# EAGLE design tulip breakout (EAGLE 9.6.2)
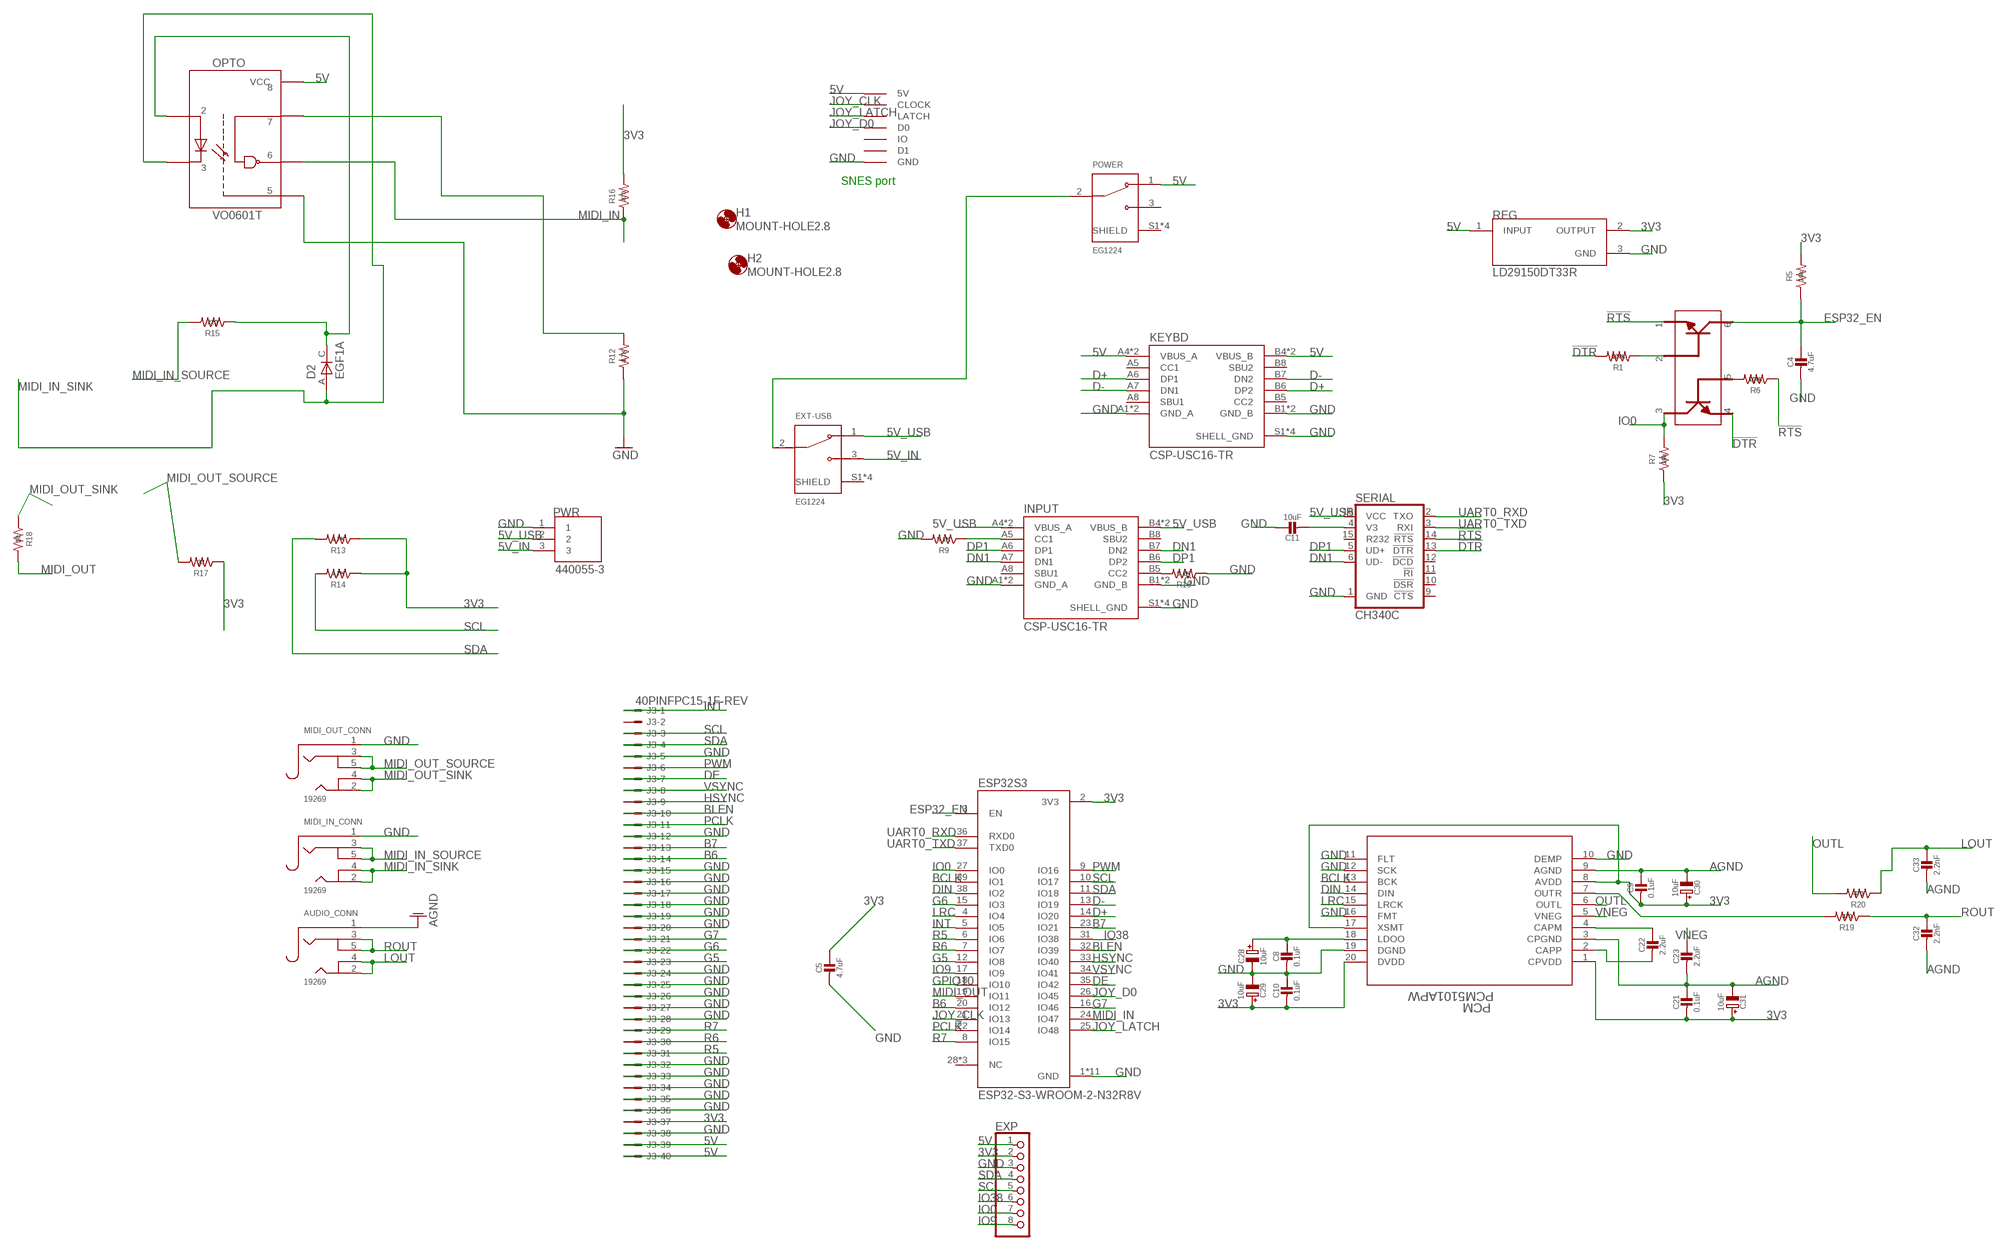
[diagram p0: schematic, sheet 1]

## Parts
AUDIO_CONN  19269  AUDIO_3.5MMJACK  [4UCONN_19269]
C4  4.7uF  CAP_CERAMIC0805-NOOUTLINE  [0805-NO]
C5  4.7uF  CAP_CERAMIC0805-NOOUTLINE  [0805-NO]
C8  0.1uF  CAP_CERAMIC0805-NOOUTLINE  [0805-NO]
C9  0.1uF  CAP_CERAMIC0805-NOOUTLINE  [0805-NO]
C10  0.1uF  CAP_CERAMIC0805-NOOUTLINE  [0805-NO]
C11  10uF  CAP_CERAMIC0805-NOOUTLINE  [0805-NO]
C21  0.1uF  CAP_CERAMIC0805-NOOUTLINE  [0805-NO]
C22  2.2uF  CAP_CERAMIC0805-NOOUTLINE  [0805-NO]
C23  2.2uF  CAP_CERAMIC0805-NOOUTLINE  [0805-NO]
C28  10uF  CAP_ELECTROLYTICPANASONIC_C  [PANASONIC_C]
C29  10uF  CAP_ELECTROLYTICPANASONIC_C  [PANASONIC_C]
C30  10uF  CAP_ELECTROLYTICPANASONIC_C  [PANASONIC_C]
C31  10uF  CAP_ELECTROLYTICPANASONIC_C  [PANASONIC_C]
C32  2.2nF  CAP_CERAMIC0805-NOOUTLINE  [0805-NO]
C33  2.2nF  CAP_CERAMIC0805-NOOUTLINE  [0805-NO]
D2  EGF1A  [DIOM449X264X300L114X135N]
ESP32S3  ESP32-S3-WROOM-2-N32R8V  [XCVR_ESP32-S3-WROOM-2-N32R8V]
EXP  PINHD-1X8BIG  [1X08-BIG]
EXT-USB  EG1224  [SW_EG1224]
H1  MOUNT-HOLE2.8  [2,8]
H2  MOUNT-HOLE2.8  [2,8]
INPUT  CSP-USC16-TR  [VALCON_CSP-USC16-TR]
J3  40PINFPC15-1F-REV  [XF2M-4015-1F-REVERSE]
KEYBD  CSP-USC16-TR  [VALCON_CSP-USC16-TR]
MIDI_IN_CONN  19269  AUDIO_3.5MMJACK  [4UCONN_19269]
MIDI_OUT_CONN  19269  AUDIO_3.5MMJACK  [4UCONN_19269]
OPTO  VO0601T  [SOIC127P610X331-8N]
PCM  PCM5101APW  [PW20_TEX]
POWER  EG1224  [SW_EG1224]
PWR  440055-3  [TE_440055-3]
R1  100k  R-US_R0805  [R0805]
R5  10k  R-US_R0805  [R0805]
R6  100k  R-US_R0805  [R0805]
R7  10k  R-US_R0805  [R0805]
R9  5.1K  R-US_R0805  [R0805]
R10  5.1K  R-US_R0805  [R0805]
R12  4.7K  R-US_R0805  [R0805]
R13  4.7K  R-US_R0805  [R0805]
R14  4.7K  R-US_R0805  [R0805]
R15  220  R-US_R0805  [R0805]
R16  470  R-US_R0805  [R0805]
R17  33  R-US_R0805  [R0805]
R18  10  R-US_R0805  [R0805]
R19  470  R-US_R0805  [R0805]
R20  470  R-US_R0805  [R0805]
REG  LD29150DT33R  [DPAK456P972X240-3N]
RESET  MBT3904DW1T1G  [SOT236]
SERIAL  CH340C  [SO016]
SNES  SNESCONN  [SNESCONN]

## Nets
3V3: C5.1 C9.2 C10.2 C21.2 C29.+ C30.+ C31.+ ESP32S3.2(3V3) EXP.2 J3.37 PCM.1(CPVDD) PCM.8(AVDD) PCM.17(XSMT) PCM.20(DVDD) R5.2 R7.1 R13.1 R14.1 R16.2 R17.1 REG.2(OUTPUT)
5V: EXP.1 J3.39 J3.40 KEYBD.A4(VBUS_A) KEYBD.A9(VBUS_A) KEYBD.B4(VBUS_B) KEYBD.B9(VBUS_B) OPTO.8(VCC) POWER.1 REG.1(INPUT) SNES.5V
5V_IN: EXT-USB.3 PWR.3
5V_USB: EXT-USB.1 INPUT.A4(VBUS_A) INPUT.A9(VBUS_A) INPUT.B4(VBUS_B) INPUT.B9(VBUS_B) PWR.2 SERIAL.16(VCC)
!DTR: R1.2 RESET.4 SERIAL.13(!DTR)
!RTS: R6.1 RESET.1 SERIAL.14(!RTS)
AGND: AUDIO_CONN.1 C9.1 C21.1 C23.2 C30.- C31.- C32.2 C33.2 PCM.3(CPGND) PCM.9(AGND)
B6: ESP32S3.20(IO12) J3.14
B7: ESP32S3.23(IO21) J3.13
BCLK: ESP32S3.39(IO1) PCM.13(BCK)
BLEN: ESP32S3.32(IO39) J3.10
D+: ESP32S3.14(IO20) KEYBD.A6(DP1) KEYBD.B6(DP2)
D-: ESP32S3.13(IO19) KEYBD.A7(DN1) KEYBD.B7(DN2)
DE: ESP32S3.35(IO42) J3.7
DIN: ESP32S3.38(IO2) PCM.14(DIN)
DN1: INPUT.A7(DN1) INPUT.B7(DN2) SERIAL.6(UD-)
DP1: INPUT.A6(DP1) INPUT.B6(DP2) SERIAL.5(UD+)
ESP32_EN: C4.1 ESP32S3.3(EN) R5.1 RESET.6
EXT-USB: EXT-USB.2 POWER.2
G5: ESP32S3.12(IO8) J3.23
G6: ESP32S3.15(IO3) J3.22
G7: ESP32S3.16(IO46) J3.21
GND: C4.2 C5.2 C8.2 C10.1 C11.1 C28.- C29.- ESP32S3.1(GND) ESP32S3.40(GND) ESP32S3.41_1(GND) ESP32S3.41_2(GND) ESP32S3.41_3(GND) ESP32S3.41_4(GND) ESP32S3.41_5(GND) ESP32S3.41_6(GND) ESP32S3.41_7(GND) ESP32S3.41_8(GND) ESP32S3.41_9(GND) EXP.3 INPUT.A1(GND_A) INPUT.A12(GND_A) INPUT.B1(GND_B) INPUT.B12(GND_B) INPUT.S1(SHELL_GND) INPUT.S2(SHELL_GND) INPUT.S3(SHELL_GND) INPUT.S4(SHELL_GND) J3.5 J3.12 J3.15 J3.16 J3.17 J3.18 J3.19 J3.20 J3.24 J3.25 J3.26 J3.27 J3.28 J3.32 J3.33 J3.34 J3.35 J3.36 J3.38 KEYBD.A1(GND_A) KEYBD.A12(GND_A) KEYBD.B1(GND_B) KEYBD.B12(GND_B) KEYBD.S1(SHELL_GND) KEYBD.S2(SHELL_GND) KEYBD.S3(SHELL_GND) KEYBD.S4(SHELL_GND) MIDI_IN_CONN.1 MIDI_OUT_CONN.1 OPTO.5(GND) PCM.10(DEMP) PCM.11(FLT) PCM.12(SCK) PCM.16(FMT) PCM.19(DGND) PWR.1 R9.2 R10.1 R12.1 REG.3(GND) SERIAL.1(GND) SNES.GND
GPIO10: ESP32S3.18(IO10)
HSYNC: ESP32S3.33(IO40) J3.9
INT: ESP32S3.5(IO5) J3.1
IO0: ESP32S3.27(IO0) EXP.7 R7.2 RESET.3
IO9: ESP32S3.17(IO9) EXP.8
IO38: ESP32S3.31(IO38) EXP.6
JOY_CLK: ESP32S3.21(IO13) SNES.CLOCK
JOY_D0: ESP32S3.26(IO45) SNES.D0
JOY_LATCH: ESP32S3.25(IO48) SNES.LATCH
LOUT: AUDIO_CONN.2 AUDIO_CONN.4 C33.1 R20.1
LRC: ESP32S3.4(IO4) PCM.15(LRCK)
MIDI_IN: ESP32S3.24(IO47) OPTO.6(VO) R16.1
MIDI_IN_SINK: D2.A MIDI_IN_CONN.2 MIDI_IN_CONN.4 OPTO.3(C)
MIDI_IN_SOURCE: MIDI_IN_CONN.3 MIDI_IN_CONN.5 R15.2
MIDI_OUT: ESP32S3.19(IO11) R18.2
MIDI_OUT_SINK: MIDI_OUT_CONN.2 MIDI_OUT_CONN.4 R18.1
MIDI_OUT_SOURCE: MIDI_OUT_CONN.3 MIDI_OUT_CONN.5 R17.2
N$1: R1.1 RESET.2
N$2: R6.2 RESET.5
N$3: INPUT.B5(CC2) R10.2
N$7: C8.1 C28.+ PCM.18(LDOO)
N$8: PCM.7(OUTR) R19.2
N$16: C22.1 PCM.4(CAPM)
N$18: C22.2 PCM.2(CAPP)
N$30: D2.C OPTO.2(A) R15.1
N$32: OPTO.7(VE) R12.2
N$38: C11.2 SERIAL.4(V3)
N$42: INPUT.A5(CC1) R9.1
OUTL: PCM.6(OUTL) R20.2
PCLK: ESP32S3.22(IO14) J3.11
PWM: ESP32S3.9(IO16) J3.6
R5: ESP32S3.6(IO6) J3.31
R6: ESP32S3.7(IO7) J3.30
R7: ESP32S3.8(IO15) J3.29
ROUT: AUDIO_CONN.3 AUDIO_CONN.5 C32.1 R19.1
SCL: ESP32S3.10(IO17) EXP.5 J3.3 R14.2
SDA: ESP32S3.11(IO18) EXP.4 J3.4 R13.2
UART0_RXD: ESP32S3.36(RXD0) SERIAL.2(TXO)
UART0_TXD: ESP32S3.37(TXD0) SERIAL.3(RXI)
VNEG: C23.1 PCM.5(VNEG)
VSYNC: ESP32S3.34(IO41) J3.8
Unconnected: ESP32S3.28(NC) ESP32S3.29(NC) ESP32S3.30(NC) EXT-USB.S1(SHIELD) EXT-USB.S2(SHIELD) EXT-USB.S3(SHIELD) EXT-USB.S4(SHIELD) INPUT.A8(SBU1) INPUT.B8(SBU2) J3.2 KEYBD.A5(CC1) KEYBD.A8(SBU1) KEYBD.B5(CC2) KEYBD.B8(SBU2) POWER.3 POWER.S1(SHIELD) POWER.S2(SHIELD) POWER.S3(SHIELD) POWER.S4(SHIELD) SERIAL.9(!CTS) SERIAL.10(!DSR) SERIAL.11(!RI) SERIAL.12(!DCD) SERIAL.15(R232) SNES.D1 SNES.IO

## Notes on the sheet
- SNES port

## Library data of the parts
AUDIO_CONN MIDI_IN_CONN MIDI_OUT_CONN = microbuilder:AUDIO_3.5MMJACK: 3.5MM Audio Jack These are normally connected as follows, from left-to right on the schematic symbol above: Tip: Left Audio Inner Ring: Right Audio Shell: Common/GND
C4 C5 C8-C11 C21-C23 C32 C33 = microbuilder:CAP_CERAMIC: Ceramic Capacitors
C28-C31 = microbuilder:CAP_ELECTROLYTIC: Electrolytic Capacitors
D2 = EGF1A:EGF1A: EGF1A Series 1 A 100 V 50 ns Surface Mount Fast Recovery Rectifier - DO-214AC Check availability; AVAILABILITY: In Stock; DESCRIPTION: Diode Standard 50 V 1A Surface Mount DO-214AC (SMA); MF: ON Semiconductor; MP: EGF1A; PACKAGE: SMA-2 ON Semiconductor; PRICE: None; PURCHASE-URL: https://pricing.snapeda.com/search/part/EGF1A/?ref=eda
ESP32S3 = ESP32-S3-WROOM-2-N32R8V:ESP32-S3-WROOM-2-N32R8V: Check availability; AVAILABILITY: In Stock; DESCRIPTION: Bluetooth, WiFi 802.11b/g/n, Bluetooth v5.0 Transceiver Module 2.4GHz PCB Trace Surface Mount; MF: Espressif Systems; MP: ESP32-S3-WROOM-2-N32R8V; PACKAGE: Package; PRICE: None; PURCHASE-URL: https://pricing.snapeda.com/search/part/ESP32-S3-WROOM-2-N32R8V/?ref=eda
EXP = adafruit:PINHD-1X8: PIN HEADER
EXT-USB POWER = EG1224:EG1224; DESCRIPTION: Slide Switch SPDT Through Hole, Right Angle; DIGI-KEY_PART_NUMBER: EG2585-ND; MF: E-Switch; MP: EG1224; PACKAGE: None; PURCHASE-URL: https://pricing.snapeda.com/search/part/EG1224/?ref=eda
H1 H2 = holes:MOUNT-HOLE: MOUNTING HOLE with drill center marker
INPUT KEYBD = CSP-USC16-TR:CSP-USC16-TR: CSP-USC16-TR Valcon USB Type C Surface Mount PCB Socket Check availability; AVAILABILITY: In Stock; DESCRIPTION: CSP-USC16-TR Valcon USB Type C Surface Mount PCB Socket; MF: Valcon; MP: CSP-USC16-TR; PACKAGE: None; PRICE: None; PURCHASE-URL: https://pricing.snapeda.com/search/part/CSP-USC16-TR/?ref=eda
J3 = adafruit:40PINFPC: OMRON FPC Connector Source : http://www.omron.com/ecb/products/pdf/fpc.pdf XF2M-4015-rev is good for connecting up 'PSP' SHARP LQ043 LCDs
OPTO = VO0601T:VO0601T: High Speed Optocoupler, 10 MBd, SOIC-8 Package; DESCRIPTION: Logic Output Optoisolator 10MBd Open Drain 4000Vrms 1 Channel 5kV/µs CMTI 8-SOIC; DIGI-KEY_PART_NUMBER: 751-1377-2-ND; MF: Vishay Semiconductors; MP: VO0601T; PACKAGE: None; PURCHASE-URL: https://pricing.snapeda.com/search/part/VO0601T/?ref=eda
PCM = pcm5101apw:PCM5101APW; COPYRIGHT: Copyright (C) 2022 Ultra Librarian. All rights reserved.; DIGI-KEY_PART_NUMBER_1: PCM5101APW-ND; MANUFACTURER_PART_NUMBER: PCM5101APW; MFR_NAME: Texas Instruments
PWR = 440055-3:440055-3; COMMENT: 440055-3; DESCRIPTION: Connector Header Through Hole, Right Angle 3 position 0.079 (2.00mm); DIGI-KEY_PART_NUMBER: A100044-ND; EU_ROHS_COMPLIANCE: Compliant; MF: TE Connectivity; MP: 440055-3; PACKAGE: None; PURCHASE-URL: https://pricing.snapeda.com/search/part/440055-3/?ref=eda
R1 R5-R7 R9 R10 R12-R20 = adafruit:R-US_: RESISTOR, American symbol
REG = LD29150DT33R:LD29150DT33R: LD29150 Series 1.5 A 3.3 V Fixed Output SMT LDO Voltage Regulator - TO-252; DESCRIPTION: Linear Voltage Regulator IC Positive Fixed 1 Output 1.5A DPAK; DIGI-KEY_PART_NUMBER: 497-1496-2-ND; MF: STMicroelectronics; MP: LD29150DT33R; PACKAGE: TO-252 STMicroelectronics; PURCHASE-URL: https://pricing.snapeda.com/search/part/LD29150DT33R/?ref=eda
RESET = MBT3904DW1T1G:MBT3904DW1T1G: Check availability; AVAILABILITY: In Stock; DESCRIPTION: Bipolar (BJT) Transistor Array 2 NPN (Dual) 40V 200mA 300MHz 150mW Surface Mount SC-88/SC70-6/SOT-363; MF: ON Semiconductor; MP: MBT3904DW1T1G; PACKAGE: SC-88-6 ON Semiconductor; PRICE: None; PURCHASE-URL: https://pricing.snapeda.com/search/part/MBT3904DW1T1G/?ref=eda
SERIAL = SparkFun-IC-Comms:CH340C; PROD_ID: IC-14038
SNES = gamepad-conn:SNESCONN

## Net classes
1 power: width 0.178 mm

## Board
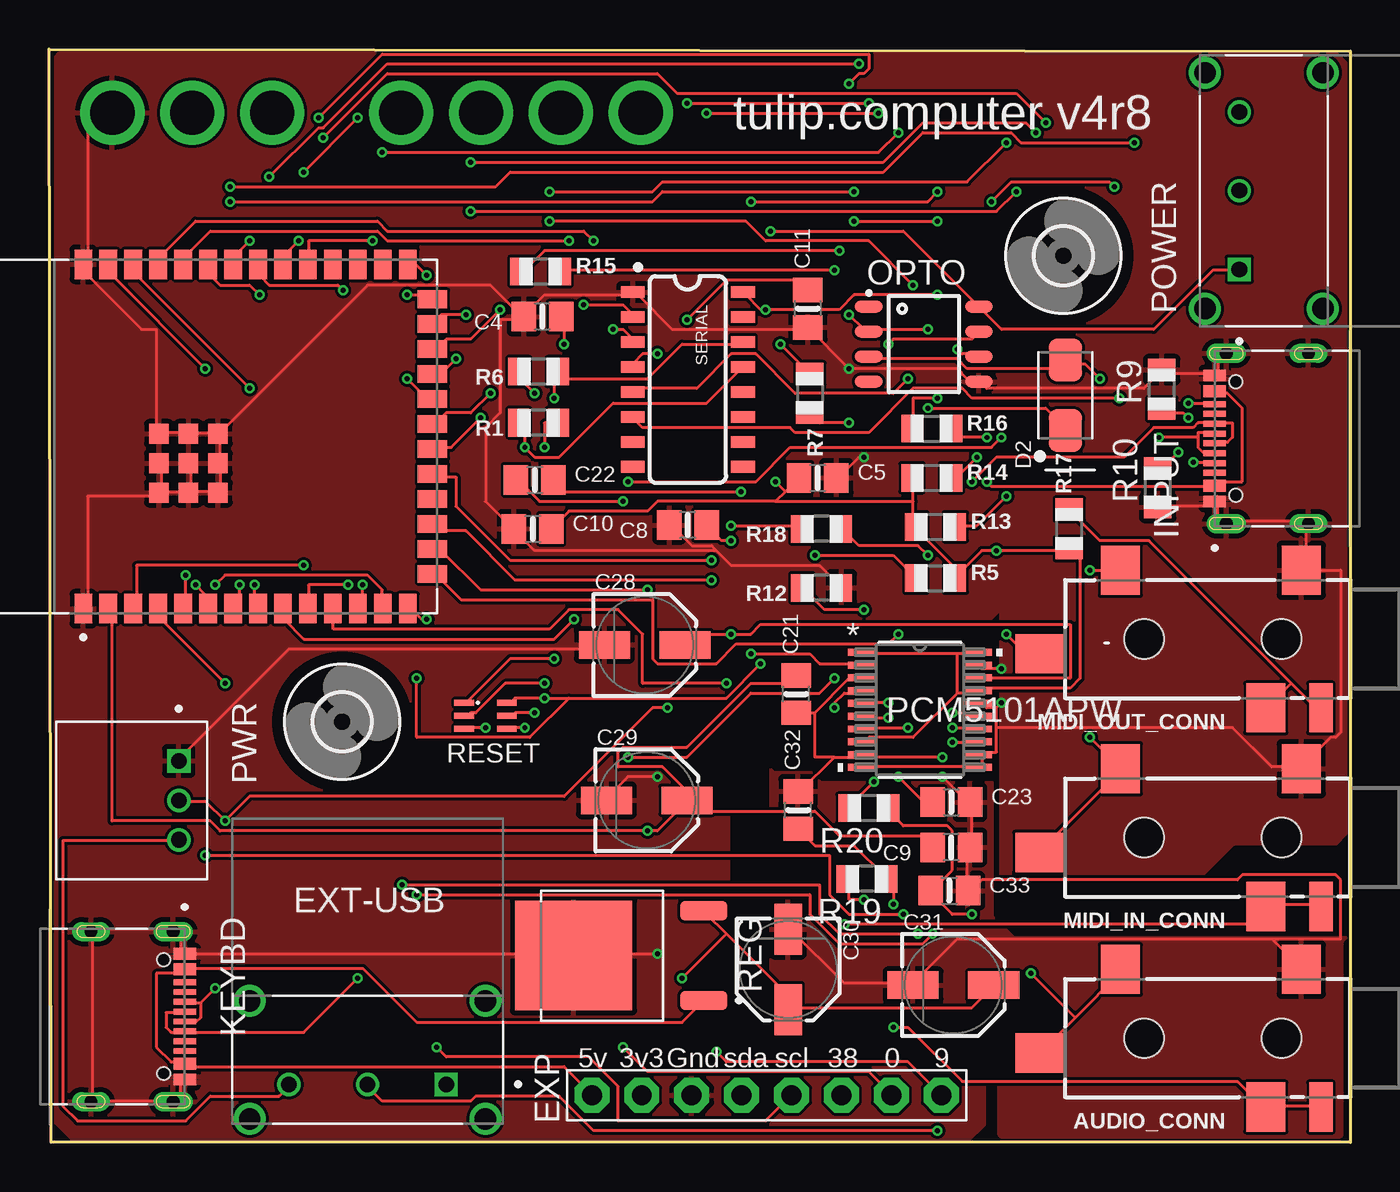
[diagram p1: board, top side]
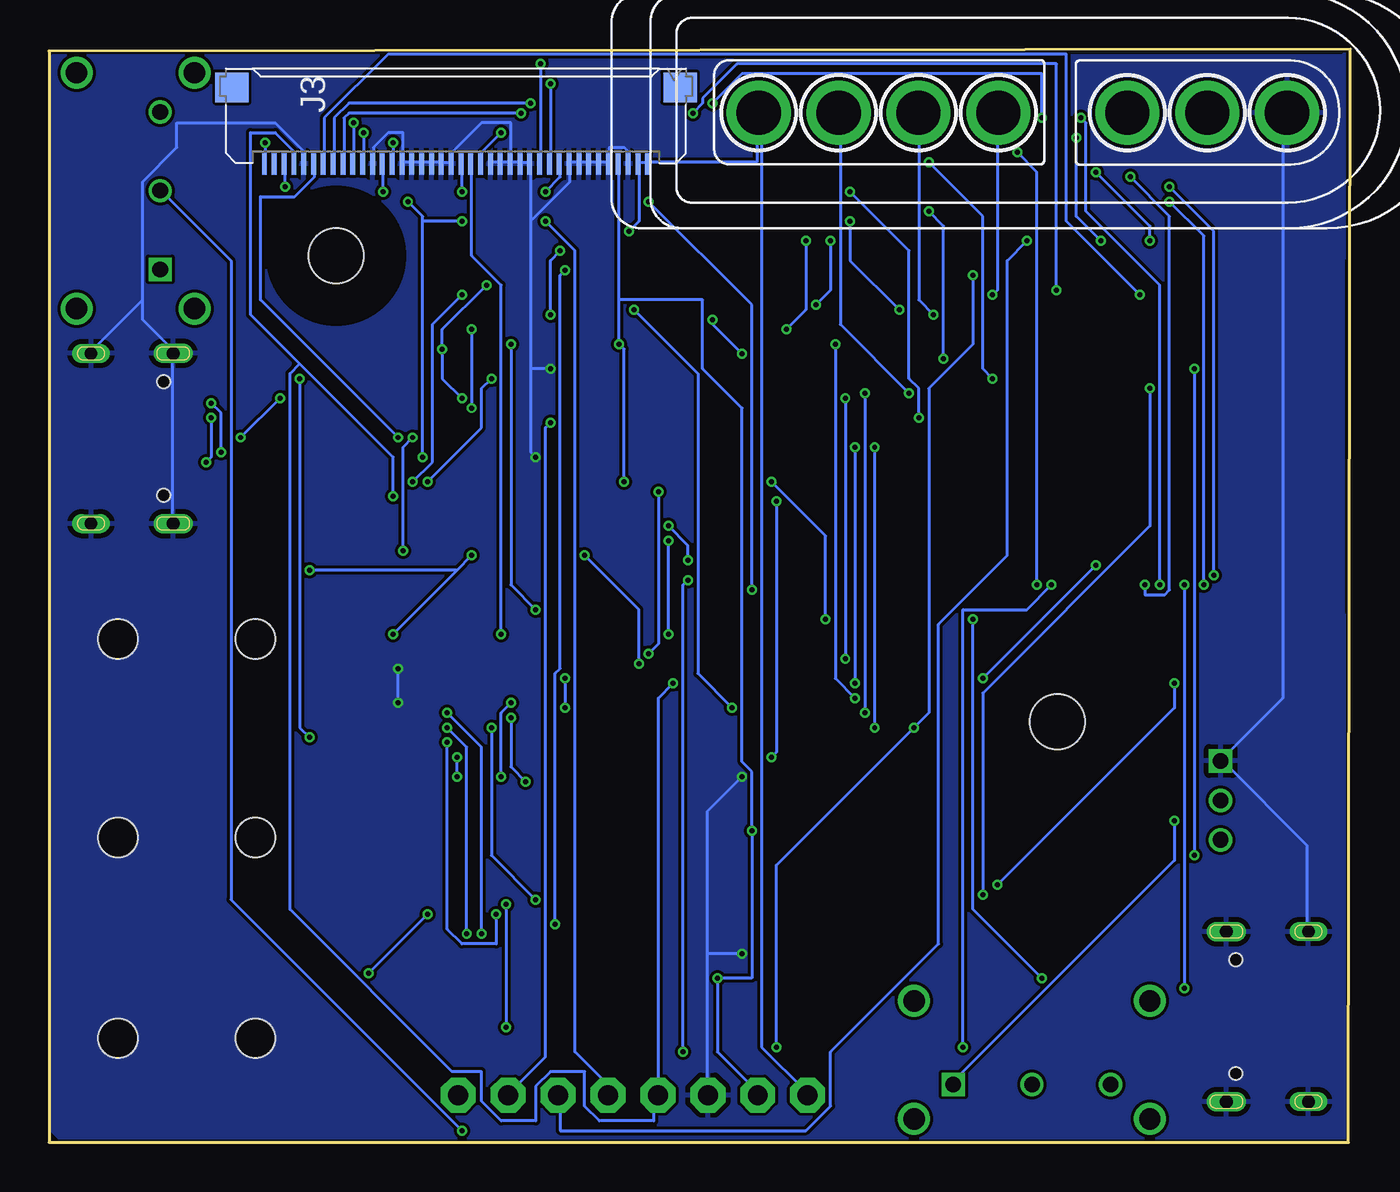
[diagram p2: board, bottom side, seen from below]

Size 66.2 x 55.6 mm. Coordinates in mm from the lower left corner, seen from the top.
Outline: 0.1,0 0,55.6 66.2,55.5 66.2,0 0.1,0
Copper layers (1*16): Top 0.035559375mm / dielectric 1.6mm / Bottom 0.035559375mm
Design rules "oshpark-2layer *": minimum track width 6mil, minimum drill 10mil, track to track 6mil, track to pad 6mil, pad to pad 6mil, via to via 6mil, smd to smd 6mil, copper to edge 0mil, drill to drill 6mil, minimum pad ring 5mil, minimum via ring 5mil, stop-mask expansion 2.5mil, vias tented up to drill 0mil, thermal gap 10mil

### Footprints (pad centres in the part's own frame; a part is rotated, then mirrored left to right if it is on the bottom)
4UCONN_19269 = smd 2 x 2.5: 1 2.5,-3.5; 2 11.7,-3.5; 3 4.3,3.5 | smd 2.5 x 2: 4 15.8,0.75 | smd 1.2 x 2.5: 5 1.5,3.5 | hole 2: 3.5,0; 10.5,0
0805-NO = smd 1.24 x 1.5: 1 -0.95,0; 2 0.95,0
PANASONIC_C = smd 2.6 x 1.4: + 2.05,0; - -2.05,0
DIOM449X264X300L114X135N = smd 2.17 x 1.69: A 1.795,0; C -1.795,0
XCVR_ESP32-S3-WROOM-2-N32R8V = smd 1.5 x 0.9: 1 -8.75,5.26; 2 -8.75,3.99; 3 -8.75,2.72; 4 -8.75,1.45; 5 -8.75,0.18; 6 -8.75,-1.09; 7 -8.75,-2.36; 8 -8.75,-3.63; 9 -8.75,-4.9; 10 -8.75,-6.17; 11 -8.75,-7.44; 12 -8.75,-8.71; 13 -8.75,-9.98; 14 -8.75,-11.25; 27 8.75,-11.25; 28 8.75,-9.98; 29 8.75,-8.71; 30 8.75,-7.44; 31 8.75,-6.17; 32 8.75,-4.9; 33 8.75,-3.63; 34 8.75,-2.36; 35 8.75,-1.09; 36 8.75,0.18; 37 8.75,1.45; 38 8.75,2.72; 39 8.75,3.99; 40 8.75,5.26 | smd 0.9 x 1.5: 15 -6.985,-12.5; 16 -5.715,-12.5; 17 -4.445,-12.5; 18 -3.175,-12.5; 19 -1.905,-12.5; 20 -0.635,-12.5; 21 0.635,-12.5; 22 1.905,-12.5; 23 3.175,-12.5; 24 4.445,-12.5; 25 5.715,-12.5; 26 6.985,-12.5 | smd 1 x 1: 41_1 -1.36,-0.09; 41_2 -2.86,-0.09; 41_3 0.14,-0.09; 41_4 -2.86,-1.59; 41_5 -1.36,-1.59; 41_6 0.14,-1.59; 41_7 -2.86,1.41; 41_8 -1.36,1.41; 41_9 0.14,1.41
1X08-BIG = drill 1.016 pad 1.778 octagon: 1 -8.89,0; 2 -6.35,0; 3 -3.81,0; 4 -1.27,0; 5 1.27,0; 6 3.81,0; 7 6.35,0; 8 8.89,0
SW_EG1224 = drill 0.79 square: 1 -4,1.25 | drill 0.79: 2 0,1.25; 3 4,1.25 | drill 1.09: S1 -6,-3; S2 6,-3; S3 6,3; S4 -6,3
2,8 = hole 2.8: 0,0
VALCON_CSP-USC16-TR = smd 0.3 x 1.14: A1 -3.35,0; A4 -2.55,0; A5 -1.25,0; A6 -0.25,0; A7 0.25,0; A8 1.25,0; A9 2.55,0; A12 3.35,0; B1 3.05,0; B4 2.25,0; B5 1.75,0; B6 0.75,0; B7 -0.75,0; B8 -1.75,0; B9 -2.25,0; B12 -3.05,0 | drill 0.65 pad 1 long: S1 -4.325,-0.59; S2 4.325,-0.59 | drill 0.65 pad 0.9 long: S3 -4.325,-4.77; S4 4.325,-4.77 | hole 0.65: -2.89,-1.07; 2.89,-1.07
XF2M-4015-1F-REVERSE = smd 1.1 x 0.25: 1 -2.54,9.75; 2 -2.54,9.25; 3 -2.54,8.75; 4 -2.54,8.25; 5 -2.54,7.75; 6 -2.54,7.25; 7 -2.54,6.75; 8 -2.54,6.25; 9 -2.54,5.75; 10 -2.54,5.25; 11 -2.54,4.75; 12 -2.54,4.25; 13 -2.54,3.75; 14 -2.54,3.25; 15 -2.54,2.75; 16 -2.54,2.25; 17 -2.54,1.75; 18 -2.54,1.25; 19 -2.54,0.75; 20 -2.54,0.25; 21 -2.54,-0.25; 22 -2.54,-0.75; 23 -2.54,-1.25; 24 -2.54,-1.75; 25 -2.54,-2.25; 26 -2.54,-2.75; 27 -2.54,-3.25; 28 -2.54,-3.75; 29 -2.54,-4.25; 30 -2.54,-4.75; 31 -2.54,-5.25; 32 -2.54,-5.75; 33 -2.54,-6.25; 34 -2.54,-6.75; 35 -2.54,-7.25; 36 -2.54,-7.75; 37 -2.54,-8.25; 38 -2.54,-8.75; 39 -2.54,-9.25; 40 -2.54,-9.75 | smd 1.5 x 1.7: M1 1.36,11.4; M2 1.36,-11.4
SOIC127P610X331-8N = smd 1.4 x 0.6: 1 -2.8,1.905; 2 -2.8,0.635; 3 -2.8,-0.635; 4 -2.8,-1.905; 5 2.8,-1.905; 6 2.8,-0.635; 7 2.8,0.635; 8 2.8,1.905
PW20_TEX = smd 1.473 x 0.356: 1 -2.921,2.925; 2 -2.921,2.275; 3 -2.921,1.625; 4 -2.921,0.975; 5 -2.921,0.325; 6 -2.921,-0.325; 7 -2.921,-0.975; 8 -2.921,-1.625; 9 -2.921,-2.275; 10 -2.921,-2.925; 11 2.921,-2.925; 12 2.921,-2.275; 13 2.921,-1.625; 14 2.921,-0.975; 15 2.921,-0.325; 16 2.921,0.325; 17 2.921,0.975; 18 2.921,1.625; 19 2.921,2.275; 20 2.921,2.925
TE_440055-3 = drill 0.8 pad 1.15 square: 1 0,0 | drill 0.8 pad 1.15: 2 2.007,0; 3 4.013,0
R0805 = smd 1.1 x 1.4: 1 -1,0; 2 1,0
DPAK456P972X240-3N = smd 2.4 x 0.98: 1 -4.2,2.28; 2 -4.2,-2.28 | smd 5.96 x 5.57: 3 2.42,0
SOT236 = smd 0.3 x 1: 1 -0.66,-1.09; 2 0,-1.09; 3 0.66,-1.09; 4 0.66,1.09; 5 0,1.09; 6 -0.66,1.09
SO016 = smd 0.6 x 1.2: 1 -4.445,-2.8; 2 -3.175,-2.8; 3 -1.905,-2.8; 4 -0.635,-2.8; 5 0.635,-2.8; 6 1.905,-2.8; 7 3.175,-2.8; 8 4.445,-2.8; 9 4.445,2.8; 10 3.175,2.8; 11 1.905,2.8; 12 0.635,2.8; 13 -0.635,2.8; 14 -1.905,2.8; 15 -3.175,2.8; 16 -4.445,2.8
SNESCONN = drill 2.25 pad 3.25: 5V 0,4.064; CLOCK 4.064,4.064; D0 12.192,4.064; D1 18.756,4.064; GND 26.884,4.064; IO 22.82,4.064; LATCH 8.128,4.064

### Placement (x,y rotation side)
AUDIO_CONN  66.2,5.3 180 top
C4  25.1,42 180 top
C5  39.1,33.8 0 top
C8  32.5,31.4 180 top
C9  45.9,15 180 top
C10  24.6,31.2 0 top
C11  38.6,42.4 90 top
C21  38,22.8 90 top
C22  24.7,33.7 0 top
C23  45.9,17.3 0 top
C28  30.3,25.3 0 top
C29  30.4,17.4 0 top
C30  37.6,8.8 270 top
C31  46,8 0 top
C32  38.1,16.9 90 top
C33  45.8,12.8 0 top
D2  51.7,38 90 top
ESP32S3  7,35.9 90 top
EXP  36.5,2.4 0 top
EXT-USB  16.2,4.2 180 top
H1  51.6,45.1 0 top
H2  14.9,21.4 0 top
INPUT  59.3,35.8 90 top
J3  45.5,52.3 90 bottom
KEYBD  6.9,6.4 270 top
MIDI_IN_CONN  66.2,15.5 180 top
MIDI_OUT_CONN  66.2,25.6 180 top
OPTO  44.5,40.6 0 top
PCM  44.3,22 0 top
POWER  61.8,48.4 90 top
PWR  6.6,19.4 270 top
R1  24.9,36.6 180 top
R5  45.1,28.7 0 top
R6  24.9,39.2 180 top
R7  38.7,38.1 270 top
R9  56.6,38.3 90 top
R10  56.4,33.3 90 top
R12  39.3,28.2 180 top
R13  45.1,31.3 0 top
R14  44.9,33.8 0 top
R15  25,44.3 0 top
R16  44.9,36.3 0 top
R17  51.9,31.2 90 top
R18  39.3,31.2 180 top
R19  41.6,13.4 180 top
R20  41.7,17 180 top
REG  29.1,9.5 180 top
RESET  22.2,21.7 270 top
SERIAL  32.5,38.8 270 top
SNES  30.1,48.3 0 bottom

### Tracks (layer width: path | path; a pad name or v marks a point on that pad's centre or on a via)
3V3  (via drill 0.25)
  Top 0.152: 46.2,24.85 47.2,24.85 PCM.20 | 46.2,24.85 41.45,24.85 PCM.1 | 46.2,22.85 43.95,20.6 41.7,20.6 41.45,20.35 PCM.8 | 46.2,22.85 47.2,22.85 PCM.17 47.45,23.1 51.95,23.1 52.45,23.6 52.45,30.1 51.95,30.1 R17.1 51.7,30.1 v48.2,30.1 47.45,30.1 46.45,29.1 | 46.2,22.85 46.2,24.85 | 43.95,32.6 43.95,31.35 R13.1 44.2,31.1 46.2,29.1 46.45,29.1 | 43.95,32.6 43.95,33.6 R14.1 | 46.45,29.1 46.2,28.85 R5.2 46.45,29.1 | v47.7,35.85 46.2,35.85 45.95,36.1 R16.2 | R7.1 v37.2,40.6 | C10.2 26.45,32.1 30.45,32.1 30.95,32.6 36.95,32.6 | C5.1 37.45,33.1 | 37.45,33.1 36.95,32.6 | 37.45,33.1 v36.95,33.6 | 36.95,32.6 43.95,32.6 | 34.45,10.6 37.45,7.6 37.45,6.85 C30.+ 37.7,6.85 46.95,6.85 47.95,7.85 C31.+ | 34.45,10.6 33.45,11.6 REG.2 | 34.45,10.6 v32.2,8.35 | C21.2 37.95,23.6 37.7,23.35 35.7,23.35 32.45,20.1 29.2,20.1 28.95,19.85 28.95,19.1 31.2,19.1 32.45,17.85 C29.+ 32.45,17.35 | 32.45,17.35 32.95,16.85 38.95,16.85 40.2,15.6 44.45,15.6 44.95,15.1 C9.2 | 32.45,17.35 30.95,15.85 v30.45,15.85 8.7,15.85 8.2,16.35 3.2,16.35 3.2,27.1 ESP32S3.2
  Bottom 0.152: v47.7,35.85 48.2,35.35 v48.2,30.1 | 37.2,42.85 v37.2,40.6 36.95,40.35 v36.95,33.6 | 37.2,42.85 37.2,49.6 J3.37 | EXP.2 30.2,2.6 32.2,4.6 v32.2,8.35 30.45,8.35 v30.45,15.85 30.45,18.85 30.95,19.35 30.95,37.35 32.95,39.35 32.95,42.85 37.2,42.85
5V  (via drill 0.25)
  Top 0.152: 6.95,3.85 6.95,4.1 KEYBD.B4 6.7,4.1 6.2,4.1 5.45,4.85 5.45,8.6 6.7,8.6 KEYBD.B9 6.95,8.6 6.95,8.85 | 6.95,8.85 15.95,8.85 18.7,6.1 32.2,6.1 33.2,7.1 REG.1 | 6.95,8.85 KEYBD.A4 | 6.95,3.85 26.2,3.85 27.45,2.6 EXP.1 | 6.95,3.85 KEYBD.A9 | POWER.1 60.45,44.35 59.2,44.35 56.2,41.35 48.45,41.35 47.45,42.35 OPTO.8 47.2,42.6 43.45,46.35 v36.7,46.35
  Bottom 0.152: 35.7,49.85 36.2,49.85 J3.39 36.2,49.6 36.2,46.85 v36.7,46.35 | 35.7,49.85 30.2,49.85 30.2,52.35 SNES.5V 29.95,52.35 29.95,4.85 27.7,2.6 EXP.1 | 35.7,49.85 J3.40
5V_IN
  Top 0.152: EXT-USB.3 12.2,2.85 11.7,2.35 8.2,2.35 6.95,1.1 1.45,1.1 0.7,1.85 0.7,15.35 6.45,15.35 PWR.3
5V_USB  (via drill 0.25)
  Top 0.152: PWR.2 6.7,17.35 7.95,17.35 v8.95,16.35 10.2,17.6 26.2,17.6 30.7,22.1 v31.45,22.1 | 59.45,38.1 59.45,38.35 INPUT.A9 | 59.45,33.6 59.45,33.35 INPUT.A4 59.2,33.35 47.95,33.35 v47.7,33.6 | v45.2,43.1 40.95,43.1 40.2,42.35 v36.45,42.35 36.2,42.35 35.45,43.1 SERIAL.16 | 59.45,38.1 59.95,38.1 60.7,37.35 60.7,33.6 59.45,33.6 | 59.45,38.1 INPUT.B4 | 59.45,33.6 INPUT.B9
  Bottom 0.152: v8.95,16.35 8.95,14.35 20.2,3.1 EXT-USB.1 | v45.2,43.1 46.7,41.6 46.7,34.6 v47.7,33.6 | v31.45,22.1 33.2,23.85 33.2,39.1 v36.45,42.35
!DTR  (via drill 0.25)
  Top 0.152: v24.2,21.1 23.45,21.1 RESET.4 | R1.2 24.2,36.6 v24.2,35.35 24.7,34.85 25.95,34.85 28.7,37.6 33.45,37.6 35.2,39.35 SERIAL.13
  Bottom 0.152: v24.2,35.35 v24.2,21.1
!RTS  (via drill 0.25)
  Top 0.152: v25.7,24.6 23.45,24.6 21.2,22.35 RESET.1 | 25.7,38.85 25.7,39.1 R6.1 25.7,38.85 | 25.7,38.85 v25.7,37.85 | 25.7,38.85 30.45,38.85 32.2,40.6 35.2,40.6 SERIAL.14
  Bottom 0.152: v25.7,37.85 v25.7,24.6
AGND  (via drill 0.25)
  Top 0.152: 38.95,21.85 40.7,23.6 41.2,23.6 PCM.3 | C21.1 38.95,21.85 | 39.95,19.6 41.2,19.6 PCM.9 41.45,19.6 v45.45,19.6 | 39.95,19.6 38.2,17.85 C32.2 | 38.95,21.85 38.95,19.6 39.95,19.6 | 62.2,10.35 63.7,8.85 AUDIO_CONN.1 | 62.2,10.35 46.2,10.35 43.95,8.1 | 43.95,8.1 40.45,8.1 37.7,10.85 C30.- | 43.95,8.1 C31.- | 62.2,10.35 65.7,10.35 65.7,13.35 65.45,13.6 60.7,13.6 60.45,13.35 47.45,13.35 46.95,12.85 C33.2 46.7,12.85 46.7,14.85 C9.1 46.95,15.1 46.95,17.1 C23.2 46.7,17.35 v45.45,18.6
  Bottom 0.152: v45.45,18.6 v45.45,19.6
  pour Top: 66,10.4 49.1,10.4 48,11.5 48,18.3 39.3,18.3 38.8,18.8 36.9,18.8 36.7,19 36.7,5.3 47.5,5.3 48.3,4.5 48.3,0.4 48.4,0.3 65.7,0.3 65.8,0.4 65.8,10.2
B6  (via drill 0.25)
  Top 0.152: v48.7,50.85 46.7,48.85 31.2,48.85 30.7,48.35 v25.45,48.35 | v21.95,36.85 20.45,35.35 19.7,35.35 ESP32S3.20
  Bottom 0.152: v48.7,50.85 48.7,49.85 J3.14 | v25.45,48.35 22.45,45.35 22.45,38.85 21.95,38.35 v21.95,36.85
B7  (via drill 0.25)
  Top 0.152: v49.2,48.35 48.2,47.35 v21.45,47.35 | v20.7,39.85 19.95,39.1 19.7,39.1 ESP32S3.23
  Bottom 0.152: v49.2,48.35 49.2,49.6 J3.13 | v21.45,47.35 20.7,46.6 v20.7,39.85
BCLK  (via drill 0.25)
  Top 0.152: v45.95,20.35 47.2,20.35 PCM.13 | v43.45,11.6 40.7,11.6 39.7,12.6 39.7,14.6 v7.95,14.6 | v7.95,39.35 3.2,44.1 3.2,44.6 ESP32S3.39
  Bottom 0.152: v45.95,20.35 45.95,10.85 45.2,10.1 43.45,10.1 v43.45,11.6 | v7.95,39.35 v7.95,14.6
BLEN  (via drill 0.25)
  Top 0.152: v50.7,51.85 49.2,53.35 31.95,53.35 30.95,54.35 17.2,54.35 v13.95,51.1 | v12.7,45.85 11.7,44.85 ESP32S3.32
  Bottom 0.152: v50.7,51.85 50.7,49.85 J3.10 | v13.95,51.1 13.95,47.1 v12.7,45.85
D+  (via drill 0.25)
  Top 0.152: KEYBD.A6 6.7,6.6 5.95,6.6 5.95,5.85 6.2,5.6 6.7,5.6 KEYBD.B6 6.95,5.6 12.95,5.6 v15.7,8.35 | v19.2,26.6 18.95,26.6 18.45,27.1 ESP32S3.14
  Bottom 0.152: v19.2,26.6 19.2,11.85 v15.7,8.35
D-  (via drill 0.25)
  Top 0.152: 7.7,7.1 7.7,6.35 7.45,6.1 6.95,6.1 KEYBD.A7 | 7.7,7.1 6.95,7.1 KEYBD.B7 | v8.45,7.85 7.7,7.1 | v8.45,28.35 8.95,28.85 16.2,28.85 16.95,28.1 16.95,27.35 ESP32S3.13
  Bottom 0.152: v8.45,28.35 v8.45,7.85
DE  (via drill 0.25)
  Top 0.152: v10.7,43.1 10.2,43.6 8.7,43.6 8.2,44.1 8.2,44.6 ESP32S3.35
  Bottom 0.152: v10.7,43.1 14.45,46.85 14.45,55.35 48.95,55.35 52.2,52.1 52.2,49.85 J3.7
DIN  (via drill 0.25)
  Top 0.152: v45.95,21.1 47.2,21.1 PCM.14 | v44.95,10.6 44.45,10.1 40.2,10.1 38.7,11.6 38.7,12.6 v18.7,12.6 | v10.2,38.35 4.45,44.1 4.45,44.6 ESP32S3.38
  Bottom 0.152: v45.95,21.1 44.95,20.1 v44.95,10.6 | v18.7,12.6 18.7,22.85 10.2,31.35 v10.2,38.35
DN1  (via drill 0.25)
  Top 0.152: 58.45,35.85 58.45,36.1 59.2,36.1 INPUT.A7 | 58.45,35.85 58.45,35.35 58.7,35.1 59.2,35.1 INPUT.B7 | v54.45,37.85 46.95,37.85 46.45,38.35 43.95,38.35 41.7,36.1 37.95,36.1 37.7,36.35 30.2,36.35 29.7,36.85 SERIAL.6 | 58.45,35.85 v56.45,35.85
  Bottom 0.152: v56.45,35.85 v54.45,37.85
DP1  (via drill 0.25)
  Top 0.152: INPUT.A6 59.45,35.6 59.95,35.6 60.2,35.85 60.2,36.6 59.45,36.6 INPUT.B6 59.2,36.6 58.45,36.6 58.2,36.35 56.2,36.35 54.7,34.85 48.2,34.85 v46.95,33.6 | v43.7,38.85 42.95,38.1 37.95,38.1 35.95,40.1 34.7,40.1 32.95,38.35 29.7,38.35 SERIAL.5
  Bottom 0.152: v43.7,38.85 44.2,38.35 44.2,36.35 v46.95,33.6
ESP32_EN  (via drill 0.25)
  Top 0.152: v26.2,40.6 26.2,41.85 C4.1 | RESET.6 23.45,22.35 23.7,22.6 v25.2,22.6 26.45,22.6 | R5.1 42.95,29.85 v38.95,29.85 | v36.2,24.35 34.45,22.6 26.45,22.6 | v12.95,29.35 4.45,29.35 4.45,27.35 ESP32S3.3 | v18.7,23.6 18.7,20.6 24.45,20.6 26.45,22.6
  Bottom 0.152: v25.2,22.6 26.2,23.6 v26.2,40.6 | v38.95,29.85 36.2,27.1 v36.2,24.35 | v18.7,23.6 v12.95,29.35
EXT-USB  (via drill 0.25)
  Top 0.152: v45.2,0.6 27.7,0.6 25.95,2.35 21.7,2.35 21.45,2.1 16.95,2.1 16.2,2.85 EXT-USB.2
  Bottom 0.152: v45.2,0.6 56.95,12.35 56.95,44.85 60.45,48.35 POWER.2
G5  (via drill 0.25)
  Top 0.152: v43.2,51.35 42.2,50.35 v16.95,50.35 | v15.95,28.35 15.95,27.35 ESP32S3.12
  Bottom 0.152: v43.2,51.35 44.2,50.35 44.2,49.85 J3.23 | v16.95,50.35 15.95,49.35 v15.95,28.35
G6  (via drill 0.25)
  Top 0.152: v43.2,25.85 42.7,25.35 34.95,25.35 33.95,24.35 30.95,24.35 30.7,24.6 30.7,27.6 20.95,27.6 19.7,28.85 ESP32S3.15
  Bottom 0.152: v43.2,25.85 43.2,43.6 44.7,45.1 44.7,49.6 J3.22
G7  (via drill 0.25)
  Top 0.152: v45.2,48.35 44.7,47.85 v35.7,47.85 | v30.45,28.1 21.95,28.1 19.95,30.1 19.7,30.1 ESP32S3.16
  Bottom 0.152: v45.2,48.35 45.2,49.6 J3.21 | v35.7,47.85 30.45,42.6 v30.45,28.1
GND  (via drill 0.25)
  Top 0.152: v30.95,18.6 29.45,18.6 28.45,17.6 C29.- | KEYBD.B1 6.95,3.35 6.95,3.1 KEYBD.A12 6.7,3.1 6.7,2.1 6.45,2.1 KEYBD.S2 6.2,2.1 2.2,2.1 | 6.95,9.6 6.95,9.85 KEYBD.A1 6.7,9.85 6.7,10.6 6.45,10.6 KEYBD.S1 6.2,10.85 2.2,10.85 KEYBD.S3 2.2,10.6 2.2,2.1 | 6.95,9.6 6.95,9.35 KEYBD.B12 | C28.- 28.2,25.1 12.2,25.1 6.7,19.6 PWR.1 | 2.2,2.1 KEYBD.S4 | 6.95,9.6 26.45,9.6 REG.3 26.7,9.6 v30.95,9.6 | ESP32S3.41_6 8.45,36.1 7.2,36.1 ESP32S3.41_3 6.95,36.1 5.7,36.1 ESP32S3.41_9 5.45,36.1 5.45,41.35 4.7,41.35 1.95,44.1 1.95,44.6 ESP32S3.40 1.95,44.85 1.95,52.35 3.2,52.35 SNES.GND | 7.2,33.1 7.2,34.35 ESP32S3.41_1 | 7.2,33.1 8.45,33.1 ESP32S3.41_4 8.7,33.1 8.7,34.35 ESP32S3.41_5 8.7,34.6 8.7,35.85 ESP32S3.41_6 | 7.2,33.1 ESP32S3.41_2 6.95,33.1 5.7,33.1 | 5.7,33.1 5.7,34.35 ESP32S3.41_8 | ESP32S3.1 1.95,27.35 1.95,32.85 5.45,32.85 ESP32S3.41_7 5.7,33.1 | PCM.10 41.45,19.1 47.2,19.1 PCM.11 47.45,19.1 47.45,19.6 PCM.12 47.45,19.85 48.2,19.85 48.2,21.1 | 48.2,22.1 47.7,22.1 47.45,22.35 PCM.16 | 48.2,21.1 48.2,22.1 | v48.45,24.1 47.45,24.1 PCM.19 | 48.2,22.1 v48.45,22.35 | 59.45,32.35 59.45,32.85 INPUT.B12 | 59.45,32.35 59.45,31.6 59.7,31.6 INPUT.S1 59.95,31.6 63.95,31.6 INPUT.S3 63.95,31.35 63.95,29.1 | 59.45,32.35 INPUT.A1 59.2,32.35 56.45,32.35 R10.1 | 63.7,19.1 65.2,20.6 65.45,20.6 65.7,20.85 65.7,29.1 63.95,29.1 | 63.95,29.1 MIDI_OUT_CONN.1 | 48.2,21.1 60.2,21.1 62.2,19.1 63.7,19.1 | 63.7,19.1 MIDI_IN_CONN.1 | v41.45,34.85 41.2,34.85 40.2,33.85 C5.2 | 33.95,30.1 33.7,30.35 32.7,30.35 31.7,31.35 C8.2 | 33.95,30.1 34.7,29.35 39.2,29.35 40.2,28.35 R12.1 | 33.95,30.1 24.7,30.1 23.7,31.1 C10.1 23.45,31.35 22.2,32.6 22.2,36.35 22.95,37.1 22.95,41.85 23.95,41.85 C4.2
  Top 0.152: 29.7,43.1 25.2,43.1 24.2,42.1 C4.2 | 29.7,43.1 29.95,43.1 31.7,41.35 38.45,41.35 C11.1 v40.7,39.35 46.2,39.35 46.7,38.85 47.2,38.85 OPTO.5 47.45,38.6 47.7,38.35 55.7,38.35 56.45,39.1 R9.2 56.7,39.1 59.2,39.1 INPUT.A12 59.45,39.1 | 29.7,43.1 SERIAL.1 | 59.45,39.1 59.45,38.85 INPUT.B1 | 59.45,39.1 59.45,40.1 59.7,40.1 INPUT.S2 | ESP32S3.41_6 8.7,36.1 16.2,43.6 22.45,43.6 23.95,42.1 C4.2
  Bottom 0.152: v30.95,18.6 32.7,16.85 32.7,9.6 | 32.7,9.6 32.7,2.6 EXP.3 | KEYBD.S3 2.2,10.85 2.2,15.1 6.45,19.35 PWR.1 6.45,19.6 3.45,22.6 3.45,52.35 SNES.GND | v30.95,9.6 32.7,9.6 | v48.45,22.35 v48.45,24.1 | 46.2,49.85 45.7,49.85 | 46.2,49.85 46.7,49.85 | 46.2,49.85 J3.19 | 46.7,49.85 47.2,49.85 | 46.7,49.85 J3.18 | 47.2,49.85 47.7,49.85 | 47.2,49.85 J3.17 | 47.7,49.85 48.2,49.85 | 47.7,49.85 J3.16 | 48.2,49.85 48.2,51.35 48.95,51.35 49.7,50.6 49.7,49.85 J3.12 | 48.2,49.85 J3.15 | 37.7,49.85 37.7,50.6 36.95,50.6 36.7,50.35 36.7,49.85 J3.38 | 37.7,49.85 38.2,49.85 | 37.7,49.85 J3.36 | 38.2,49.85 38.7,49.85 | 38.2,49.85 J3.35 | 38.7,49.85 39.2,49.85 | 38.7,49.85 J3.34 | 39.2,49.85 39.7,49.85 J3.32 39.7,49.6 39.7,48.85 41.7,46.85 | 39.2,49.85 J3.33 | 42.2,49.85 41.7,49.85 J3.28 41.7,49.6 41.7,46.85 | 42.2,49.85 42.7,49.85 | 42.2,49.85 J3.27 | 42.7,49.85 43.2,49.85 | 43.2,49.85 43.7,49.85 J3.24 | 43.2,49.85 J3.25 | v41.45,34.85 41.7,35.1 41.7,39.35 | 41.7,46.85 41.7,39.35 | 45.7,49.85 45.7,50.35 44.2,51.85 42.7,51.85 42.7,49.85 | 45.7,49.85 J3.20 | 42.7,49.85 J3.26 | 61.45,42.85 61.45,41.85 59.95,40.35 INPUT.S2 59.95,40.1 59.95,31.6 INPUT.S1 | 61.45,42.85 61.45,48.85 59.7,50.6 59.7,51.85 54.7,51.85 53.2,50.35 53.2,49.85 J3.5 | 61.45,42.85 63.95,40.35 INPUT.S4 | v40.7,39.35 41.7,39.35
  pour Top: 0.3,55.2 0.3,1 1.2,0.1 46.8,0.1 47.6,0.9 47.6,4.7 47.4,4.9 35,4.9 34.6,5.3 34.6,24.3 36.1,25.8 47.1,25.8 48.4,27.1 48.4,12.8 49.4,11.8 56.9,11.8 60.3,15.2 65.5,15.2 66,15.7 66,54.9 65.5,55.4 0.5,55.4
  pour Bottom: 0.3,55.4 0.3,0.2 65.7,0.2 66.1,0.6 66.1,55.2 66,55.3 0.4,55.3
HSYNC  (via drill 0.25)
  Top 0.152: v33.45,52.35 v42.2,52.35 | v14.95,43.35 14.7,43.6 11.2,43.6 10.7,44.1 10.7,44.6 ESP32S3.33
  Bottom 0.152: v42.2,52.35 50.95,52.35 51.2,52.1 51.2,49.85 J3.9 | v33.45,52.35 32.95,52.85 32.95,53.1 31.2,54.85 14.95,54.85 v14.95,43.35
INT  (via drill 0.25)
  Top 0.152: v55.2,50.85 49.45,50.85 48.95,51.35 44.45,51.35 42.45,49.35 23.45,49.35 22.7,48.6 v9.2,48.6 | v6.95,28.85 6.95,27.35 ESP32S3.5
  Bottom 0.152: v55.2,50.85 55.2,49.85 J3.1 | v9.2,48.6 6.95,46.35 v6.95,28.85
IO0  (via drill 0.25)
  Top 0.152: v22.2,21.1 21.2,21.1 RESET.3 | v19.2,44.1 18.7,44.6 18.45,44.6 ESP32S3.27 | R7.2 39.2,36.6 v40.7,36.6 | v29.2,4.85 30.45,3.6 41.7,3.6 42.7,2.6 EXP.7
  Bottom 0.152: v19.2,44.1 19.2,40.6 21.45,38.35 21.45,21.85 v22.2,21.1 29.2,14.1 v29.2,4.85 | v40.7,36.6 40.95,36.35 40.95,4.35 42.7,2.6 EXP.7
IO9  (via drill 0.25)
  Top 0.152: v33.7,28.6 23.7,28.6 21.2,31.1 19.95,31.1 19.7,31.35 ESP32S3.17 | v33.95,4.6 34.45,4.1 43.7,4.1 45.2,2.6 EXP.8
  Bottom 0.152: v33.7,28.6 33.95,28.35 v33.95,4.6
IO38  (via drill 0.25)
  Top 0.152: v16.45,45.85 13.2,45.85 13.2,44.85 ESP32S3.31
  Bottom 0.152: v16.45,45.85 17.45,44.85 17.45,29.85 20.95,26.35 20.95,10.1 26.45,4.6 26.45,1.85 27.7,0.6 40.2,0.6 40.2,2.35 EXP.6
JOY_CLK  (via drill 0.25)
  Top 0.152: v22.45,38.1 21.45,37.1 20.2,37.1 19.7,36.6 ESP32S3.21
  Bottom 0.152: v22.45,38.1 25.95,41.6 25.95,52.35 SNES.CLOCK
JOY_D0  (via drill 0.25)
  Top 0.152: v18.2,43.1 19.45,43.1 ESP32S3.26
  Bottom 0.152: v18.2,43.1 17.95,43.35 17.95,52.35 SNES.D0
JOY_LATCH  (via drill 0.25)
  Top 0.152: v21.2,42.1 19.95,42.1 19.7,41.85 ESP32S3.25
  Bottom 0.152: v21.2,42.1 21.95,42.85 21.95,52.35 SNES.LATCH
LOUT  (via drill 0.25)
  Top 0.152: R20.1 42.7,16.85 43.45,16.1 45.7,16.1 45.95,15.85 45.95,13.85 44.95,12.85 C33.1 44.95,12.6 45.95,11.6 v46.95,11.6 | 52.2,6.35 54.45,8.6 AUDIO_CONN.2 | 52.2,6.35 AUDIO_CONN.4 | 52.2,6.35 v49.95,8.6
  Bottom 0.152: v49.95,8.6 v46.95,11.6
LRC  (via drill 0.25)
  Top 0.152: v45.95,21.85 47.2,21.85 PCM.15 | v44.2,10.6 40.2,10.6 39.2,11.6 39.2,13.1 v17.95,13.1 | v8.95,23.35 5.7,26.6 5.7,27.1 ESP32S3.4
  Bottom 0.152: v45.95,21.85 44.2,20.1 v44.2,10.6 | v17.95,13.1 8.95,22.1 v8.95,23.35
MIDI_IN  (via drill 0.25)
  Top 0.152: v45.2,37.85 43.95,37.85 43.95,36.35 R16.1 | v46.2,40.35 46.45,40.1 47.2,40.1 OPTO.6 | v22.95,42.35 21.45,40.85 20.2,40.85 19.7,40.35 ESP32S3.24 | v25.45,46.85 35.45,46.85 36.45,45.85 41.7,45.85 v43.95,43.6
  Bottom 0.152: v45.2,37.85 46.2,38.85 v46.2,40.35 46.2,41.35 v43.95,43.6 | v22.95,42.35 25.45,44.85 v25.45,46.85
MIDI_IN_SINK  (via drill 0.25)
  Top 0.152: MIDI_IN_CONN.4 50.45,14.85 54.45,18.85 MIDI_IN_CONN.2 54.45,19.1 v52.95,20.6 | 51.7,39.6 51.45,39.35 46.7,39.35 46.2,39.85 41.7,39.85 OPTO.3 | v53.45,38.85 52.7,39.6 51.7,39.6 | 51.7,39.6 D2.A
  Bottom 0.152: v52.95,20.6 53.45,21.1 v53.45,38.85
MIDI_IN_SOURCE  (via drill 0.25)
  Top 0.152: v39.95,44.35 26.2,44.35 R15.2 | v40.45,11.1 60.95,11.1 61.7,11.85 MIDI_IN_CONN.3 61.95,12.1 64.7,12.1 MIDI_IN_CONN.5
  Bottom 0.152: v39.95,44.35 40.2,44.1 40.2,24.1 40.45,23.85 v40.45,11.1
MIDI_OUT  (via drill 0.25)
  Top 0.152: v34.7,31.35 38.2,31.35 R18.2 | v33.7,29.6 23.45,29.6 20.7,32.35 20.7,33.85 19.7,33.85 ESP32S3.19
  Bottom 0.152: v34.7,31.35 33.7,30.35 v33.7,29.6
MIDI_OUT_SINK  (via drill 0.25)
  Top 0.152: v44.7,29.85 44.2,30.35 41.2,30.35 40.45,31.1 R18.1 | v48.7,25.85 49.7,24.85 MIDI_OUT_CONN.4 | v52.95,29.1 MIDI_OUT_CONN.2
  Bottom 0.152: v48.7,25.85 45.45,29.1 | 45.45,29.1 v44.7,29.85 | 45.45,29.1 v52.95,29.1
MIDI_OUT_SOURCE
  Top 0.152: 63.2,23.35 64.45,22.1 MIDI_OUT_CONN.5 | 63.2,23.35 55.95,30.6 53.45,30.6 51.95,32.1 R17.2 | 63.2,23.35 61.95,22.1 MIDI_OUT_CONN.3
N$1  (via drill 0.25)
  Top 0.152: v25.2,23.35 23.2,23.35 21.7,21.85 21.45,21.85 21.2,21.6 RESET.2 | v25.2,35.35 25.2,36.6 R1.1
  Bottom 0.152: v25.2,35.35 v25.2,23.35
N$2  (via drill 0.25)
  Top 0.152: v24.7,21.85 23.7,21.85 23.45,21.6 RESET.5 | v24.7,38.1 23.7,39.1 R6.2
  Bottom 0.152: v24.7,38.1 v24.7,21.85
N$3  (via drill 0.25)
  Top 0.152: v57.95,37.6 59.2,37.6 INPUT.B5 | v57.45,35.1 56.7,34.35 56.45,34.35 R10.2
  Bottom 0.152: v57.95,37.6 57.45,37.1 v57.45,35.1
N$7  (via drill 0.25)
  Top 0.152: PCM.18 47.45,23.6 51.95,23.6 51.95,26.35 36.2,26.35 35.7,25.85 v34.7,25.85 32.95,25.85 32.45,25.35 C28.+ | v34.7,30.6 34.2,30.6 33.45,31.35 C8.1
  Bottom 0.152: v34.7,25.85 v34.7,30.6
N$8  (via drill 0.25)
  Top 0.152: v41.45,12.35 40.7,12.35 40.7,13.35 R19.2 | v43.7,21.1 41.45,21.1 PCM.7
  Bottom 0.152: v41.45,12.35 43.7,14.6 v43.7,21.1
N$16  (via drill 0.25)
  Top 0.152: v39.95,22.1 39.95,22.35 40.45,22.85 41.2,22.85 PCM.4 | v39.95,23.6 39.2,22.85 35.7,22.85 32.45,19.6 v29.45,19.6 | v29.2,32.6 24.95,32.6 23.95,33.6 C22.1
  Bottom 0.152: v39.95,23.6 v39.95,22.1 | v29.45,19.6 29.2,19.85 v29.2,32.6
N$18  (via drill 0.25)
  Top 0.152: v35.7,24.85 38.7,24.85 39.2,24.35 41.2,24.35 PCM.2 | v35.2,33.1 26.2,33.1 25.7,33.6 C22.2
  Bottom 0.152: v35.7,24.85 35.2,25.35 v35.2,33.1
N$30  (via drill 0.25)
  Top 0.152: v40.2,45.35 25.2,45.35 24.2,44.35 R15.1 | v40.7,42.1 41.45,41.35 41.7,41.35 | v44.7,37.35 50.7,37.35 51.7,36.35 D2.C | 41.7,41.35 v44.7,41.35 | 41.7,41.35 OPTO.2
  Bottom 0.152: v40.2,45.35 40.7,44.85 v40.7,42.1 | v44.7,41.35 v44.7,37.35
N$32  (via drill 0.25)
  Top 0.152: v41.45,27.1 39.45,27.1 38.45,28.1 R12.2 | v42.7,40.6 42.95,40.85 46.95,40.85 47.2,41.1 OPTO.7
  Bottom 0.152: v41.45,27.1 42.7,28.35 v42.7,40.6
N$38  (via drill 0.25)
  Top 0.152: v30.95,40.1 30.2,40.1 29.7,39.6 SERIAL.4 | v32.45,41.85 34.45,43.85 37.95,43.85 38.45,43.35 C11.2
  Bottom 0.152: v30.95,40.1 32.45,41.6 v32.45,41.85
N$42  (via drill 0.25)
  Top 0.152: v58.2,34.6 59.2,34.6 INPUT.A5 | v57.95,36.85 57.7,37.1 56.7,37.1 R9.1
  Bottom 0.152: v58.2,34.6 57.95,34.85 v57.95,36.85
OUTL  (via drill 0.25)
  Top 0.152: v41.95,18.35 40.7,17.1 R20.2 | v42.7,21.6 41.45,21.6 PCM.6
  Bottom 0.152: v41.95,18.35 42.7,19.1 v42.7,21.6
PCLK  (via drill 0.25)
  Top 0.152: v50.2,51.35 49.7,51.85 44.45,51.85 42.45,49.85 v21.45,49.85 | v18.2,38.85 19.2,37.85 19.45,37.85 ESP32S3.22
  Bottom 0.152: v50.2,51.35 50.2,49.85 J3.11 | v21.45,49.85 18.7,47.1 18.7,39.35 v18.2,38.85
PWM  (via drill 0.25)
  Top 0.152: v48.45,35.85 47.95,35.35 37.7,35.35 35.95,33.6 v29.45,33.6 | v26.7,26.6 25.7,25.6 12.95,25.6 11.95,26.6 11.95,27.1 ESP32S3.9
  Bottom 0.152: v48.45,35.85 55.45,42.85 55.45,48.1 53.7,48.1 52.7,49.1 52.7,49.6 J3.6 | v29.45,33.6 26.7,30.85 v26.7,26.6
R5  (via drill 0.25)
  Top 0.152: v40.95,48.35 31.2,48.35 30.7,47.85 v9.2,47.85 | v7.45,28.35 7.95,27.85 7.95,27.35 ESP32S3.6
  Bottom 0.152: v40.95,48.35 40.2,49.1 40.2,49.6 J3.31 | v9.2,47.85 7.45,46.1 v7.45,28.35
R6  (via drill 0.25)
  Top 0.152: v40.7,53.85 41.2,54.35 41.45,54.35 41.7,54.6 41.7,55.35 16.95,55.35 v13.7,52.1 | v9.7,28.35 9.7,27.35 9.45,27.35 ESP32S3.7
  Bottom 0.152: v40.7,53.85 40.7,49.85 J3.30 | v13.7,52.1 13.45,51.85 13.45,47.35 9.7,43.6 v9.7,28.35
R7  (via drill 0.25)
  Top 0.152: v41.2,54.85 17.2,54.85 13.95,51.6 13.7,51.6 v11.2,49.1 | v10.45,28.35 10.45,27.35 ESP32S3.8
  Bottom 0.152: v41.2,54.85 41.2,49.85 J3.29 | v11.2,49.1 9.2,47.1 9.2,28.1 9.45,27.85 10.45,27.85 v10.45,28.35
ROUT  (via drill 0.25)
  Top 0.152: AUDIO_CONN.5 64.7,1.85 61.95,1.85 AUDIO_CONN.3 61.7,1.85 60.45,3.1 46.45,3.1 43.7,5.85 v42.95,5.85 | C32.1 38.95,15.1 40.95,15.1 42.45,13.6 R19.1 42.7,13.35 42.95,13.35 v42.95,12.1
  Bottom 0.152: v42.95,12.1 v42.95,5.85
SCL  (via drill 0.25)
  Top 0.152: v54.2,48.6 53.95,48.85 48.95,48.85 v47.95,47.85 | v47.2,34.85 46.2,33.85 45.95,33.85 R14.2 | v15.2,28.35 13.2,28.35 13.2,27.35 ESP32S3.10 | v19.7,4.85 20.2,4.35 27.45,4.35 28.95,2.85 28.95,1.1 36.45,1.1 37.7,2.35 EXP.5 | v40.95,46.85 v45.2,46.85
  Bottom 0.152: v54.2,48.6 54.2,49.6 J3.3 | v47.95,47.85 47.2,47.1 47.2,46.85 | v47.2,34.85 47.2,46.85 | v15.2,28.35 16.45,27.1 19.7,27.1 v19.7,4.85 | v45.2,46.85 47.2,46.85 | v40.95,46.85 39.45,45.35 39.45,4.6 37.95,3.1 37.95,2.6 EXP.5
SDA  (via drill 0.25)
  Top 0.152: v48.7,32.85 47.2,31.35 46.2,31.35 R13.2 | v34.45,23.35 30.2,23.35 30.2,25.85 28.95,27.1 26.45,27.1 25.45,26.1 14.45,26.1 14.45,27.1 ESP32S3.11
  Bottom 0.152: 53.45,39.6 48.7,34.85 v48.7,32.85 | 53.45,39.6 55.95,42.1 55.95,51.35 54.7,51.35 53.7,50.35 53.7,49.85 J3.4 | v34.45,23.35 35.2,22.6 35.2,2.6 EXP.4 35.45,2.35 35.45,1.1 38.2,1.1 38.95,1.85 38.95,3.6 40.7,3.6 41.45,2.85 41.45,1.1 43.2,1.1 44.2,2.1 44.2,3.6 45.7,3.6 53.95,11.85 53.95,39.1 53.45,39.6
UART0_RXD  (via drill 0.25)
  Top 0.152: v27.2,42.6 29.2,42.6 29.7,42.1 SERIAL.2 | v26.45,45.85 17.2,45.85 16.7,46.35 8.2,46.35 6.7,44.85 ESP32S3.36
  Bottom 0.152: v27.2,42.6 26.45,43.35 v26.45,45.85
UART0_TXD  (via drill 0.25)
  Top 0.152: v28.7,41.35 29.2,41.35 29.7,40.85 SERIAL.3 | v27.7,45.85 27.2,46.35 17.2,46.35 16.7,46.85 7.45,46.85 5.45,44.85 ESP32S3.37
  Bottom 0.152: v28.7,41.35 27.7,42.35 v27.7,45.85
VNEG  (via drill 0.25)
  Top 0.152: v42.7,22.35 41.45,22.35 PCM.5 | v43.2,18.6 44.45,17.35 44.95,17.35 C23.1
  Bottom 0.152: v42.7,22.35 43.2,21.85 v43.2,18.6
VSYNC  (via drill 0.25)
  Top 0.152: v32.45,52.85 v41.7,52.85 | v12.95,49.35 v15.7,52.1 | v10.2,45.85 9.2,44.85 ESP32S3.34
  Bottom 0.152: v41.7,52.85 50.95,52.85 51.7,52.1 51.7,49.85 J3.8 | v32.45,52.85 30.95,54.35 15.7,54.35 v15.7,52.1 | v12.95,49.35 10.2,46.6 v10.2,45.85

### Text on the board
tNames: tulip.computer v4r8 | RESET | 5v | 3v3 | Gnd | sda | scl | 38 | 0 | 9
tValues: Close
Measures: All dimensions in inches | Units: Inches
